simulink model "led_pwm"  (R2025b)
settings: Solver=VariableStepAuto  StartTime=0.0  StopTime=10.0  RelTol=1e-3
libraries: arduinolib x1, simulink x1

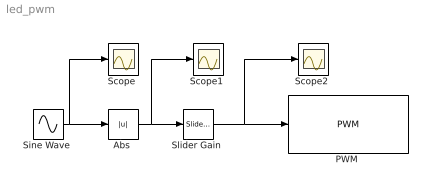
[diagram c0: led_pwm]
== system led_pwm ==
  "Abs " : Abs
  "PWM " : arduinolib/PWM  pinNumber=9  frequencyType=Default  desiredFrequency=490.2  achievableFrequency=490.2
  "Scope " : Scope
  "Scope1 " : Scope
  "Scope2 " : Scope
  "Sine Wave " : Sin  SineType=Sample based  Samples=300  SampleTime=0.01
  "Slider Gain " : simulink/Math Operations/Slider Gain  gain=130.050  low=0  high=255
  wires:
  "Sine Wave "/1 -> "Scope "/1, "Abs "/1
  "Abs "/1 -> "Slider Gain "/1, "Scope1 "/1
  "Slider Gain "/1 -> "Scope2 "/1, "PWM "/1
